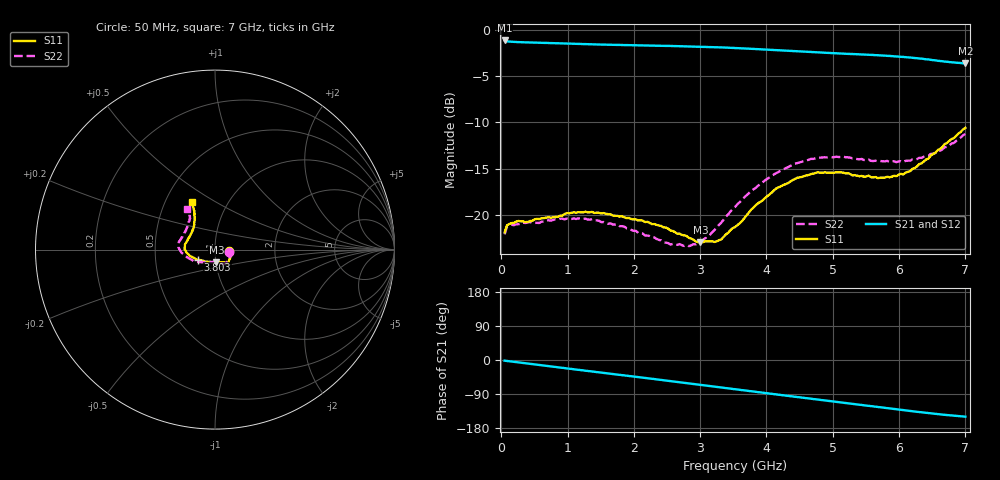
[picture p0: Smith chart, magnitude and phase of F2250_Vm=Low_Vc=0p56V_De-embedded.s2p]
! Integrated Device Technology
! Corporate Headquarters
! 6024 Silver Creek Valley Road
! San Jose, CA 95138  USA
! Phone:  1-408-284-8200
! Toll Free:  1-800-223-1366
! Webpage:  http://www.idt.com/
! Timing and RF Division
! 515 Groton Road, Suite 102
! Westford, MA 01886-6024
! Device:  F2250
! Description: Voltage Variable RF Attenuator
! Frequency:  50.0 -  6000.00 MHz
! Package:  3x3 mm Thin QFN Plastic Package: 16 pin
! Ports:  2 RF, 3 DC
!  Pin  1  = GND
!  Pin  2  = NC
!  Pin  3  = RF1  = Port 1
!  Pin  4  = NC
!  Pin  5  = GND
!  Pin  6  = GND
!  Pin  7  = GND
!  Pin  8  = GND
!  Pin  9  = NC
!  Pin 10  = RF2  = Port 2
!  Pin 11  = NC
!  Pin 12  = GND
!  Pin 13  = GND
!  Pin 14  = VCNTRL
!  Pin 15  = VDD
!  Pin 16  = VMODE
! Vcntrl:  0.560 Volts
! Vmode:  +0.000 Volts
! Vdd:  +3.30  Volts
! Current:  1.136 mA
! Data:  The device was measured on a the F2250 evaluation board which has
!  individual transmission lines to the RF pins.  Data was collected
!  using a calibrated network analyzer.  The evaluation board was
!  de-embedded using a TRL calibration technique.
!  The reference plane is the edge of the package pin.
! Misc:  SN 10
!  Action Tracker AT0258
! Date Measured:  2014-11-26
! Date:  2015-10-15  MJV
! Note:
!  Integrated Device Technology supplies this data as a sample of measured
!  data at the package pin for this product.  Your particular data for this
!  product may vary.
!  Data was taken at 25 degrees C.
!  Integrated Device Technology reserves the right to change this data at anytime.
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# GHz S dB R 50
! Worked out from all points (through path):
!   201 points, 50 MHz to 7 GHz, reference 50 ohm
!   highest |S21| = -1.17 dB at 50 MHz (marker M1); lowest = -3.7 dB at 7 GHz (marker M2)
!   group delay of S21, straight-line fit = 60.1 ps
!   lowest |S11| = -23.0 dB at 3.004 GHz (marker M3), VSWR 1.15, Z = 50.3 - j7.13 ohm
!   |S11| at or under -10 dB: start of sweep to end of sweep
!   |S22| runs from -23.4 to -11.3 dB; largest |S21 - S12| = 0.00042
!   S11 on the Smith chart (normalised r, x): 50 MHz: 1.17, -0.02; 3.803 GHz: 0.82, -0.09; 7 GHz: 0.68, +0.39
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0.05  -21.89 -6.8  -1.17 -1.8  -1.17 -1.8  -22.11 -7.9
0.08475  -21.13 -6.9  -1.26 -2.5  -1.26 -2.5  -21.29 -7.4
0.15425  -20.90 -9.0  -1.31 -4.0  -1.31 -4.0  -21.07 -9.2
0.71025  -20.25 -30.7  -1.45 -16.2  -1.44 -16.2  -20.58 -34.0
1.2315  -19.74 -46.6  -1.56 -27.4  -1.56 -27.4  -20.44 -54.0
1.75275  -20.11 -53.4  -1.66 -38.5  -1.65 -38.5  -21.02 -63.3
2.37825  -21.16 -55.8  -1.74 -51.8  -1.74 -51.8  -22.71 -70.9
2.552  -21.70 -59.1  -1.76 -55.6  -1.76 -55.6  -23.21 -76.8
2.83  -22.50 -70.2  -1.81 -61.7  -1.81 -61.7  -23.38 -92.7
3.00375  -22.98 -83.3  -1.85 -65.6  -1.84 -65.6  -22.83 -105.8
3.14275  -22.85 -94.2  -1.88 -68.6  -1.87 -68.6  -22.20 -117.1
3.3165  -22.66 -112.5  -1.92 -72.5  -1.92 -72.5  -20.85 -128.9
3.525  -21.32 -130.4  -1.98 -77.2  -1.99 -77.2  -19.15 -141.0
3.803  -19.21 -149.1  -2.08 -83.3  -2.09 -83.4  -17.25 -153.8
4.1505  -17.13 -163.7  -2.22 -91.0  -2.22 -91.0  -15.48 -167.7
4.7065  -15.54 -179.7  -2.44 -103.0  -2.44 -103.0  -13.96 178.2
5.15825  -15.45 169.3  -2.60 -112.7  -2.60 -112.7  -13.72 168.5
5.85325  -15.95 145.5  -2.84 -127.6  -2.84 -127.6  -14.29 152.8
6.166  -15.29 133.5  -3.01 -134.4  -3.01 -134.4  -14.15 143.7
6.444  -13.92 123.9  -3.22 -140.2  -3.22 -140.3  -13.62 134.2
6.82625  -11.71 117.2  -3.54 -146.9  -3.54 -146.9  -12.24 126.0
7  -10.60 116.3  -3.66 -149.6  -3.66 -149.6  -11.26 124.5
